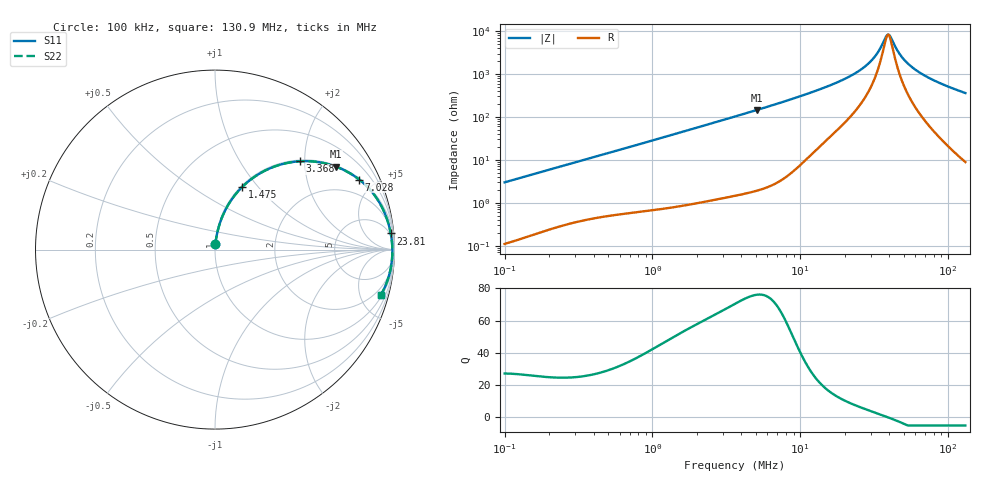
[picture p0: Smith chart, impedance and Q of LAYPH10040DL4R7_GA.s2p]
! LAYPH10040DL4R7_GA  S-PARAMETER MODEL  ( General Type )
! Model Generated by TAIYO YUDEN Corporation (http://www.ty-top.com)
! Version 1.0
! TAIYO YUDEN Control No. 180920NI43SB-FBB
! Copyright(c) 2018 TAIYO YUDEN CO.,LTD. All Rights Reserved.
! Product Description (link to TY-COMPAS)
! https://ds.yuden.co.jp/TYCOMPAS/or/detail?pn=LAYPH10040DL4R7NGA&u=M
! Products Name : Inductors
! Characteristics :
!  Inductance : 4.7 uH , SRF(min) : -Hz , DC Resistance(max) : 0.025 Ohm
!  Rated Current : Saturation :5.2 A , Temp Rise : 2.7 A (25 degC)
!  Case Size : 10.1 x 10.0 / 0.398 x 0.394 [mm/inch] , Thickness : 4 / 0.157 [mm/inch]
!  (Conditions: Temperature = 25 degC , DC Bias Current/Voltage = 0A / 0V)
! External Node Assignments :
!  1  o---GGG---o  2
! GND o---------o GND
! Frequency Range : 0.1MHz  -  130.914307MHz  [ 402 STEP ]
# MHz S RI R 50
! Freq[MHz].  S11 Real  S11 Imag  S21 Real  S21 Imag  S12 Real  S12 Imag  S22 Real  S22 Imag
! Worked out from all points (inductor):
!   401 points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, 100 kHz to 130.9 MHz, reference 50 ohm
!   read as one part in series: L = 4.73 uH near 103.7 kHz
!   highest Q = 76.1 at 5.088 MHz (marker M1), where L = 4.53 uH
!   self-resonance near 38.65 MHz
!   S11 on the Smith chart (normalised r, x): 100 kHz: 1.00, +0.06; 1.475 MHz: 1.02, +0.83; 3.368 MHz: 1.03, +1.90; 7.028 MHz: 1.06, +4.08; 23.81 MHz: 4, +21; 130.9 MHz: 1.18, -7.19
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0.1  0.00198 0.0298  0.998 -0.0298  0.998 -0.0298  0.00198 0.0298
0.332733  0.0128 0.0946  0.9872 -0.0946  0.9872 -0.0946  0.0128 0.0946
0.623493  0.0354 0.17  0.9646 -0.17  0.9646 -0.17  0.0354 0.17
1.10711  0.0941 0.2809  0.9059 -0.2809  0.9059 -0.2809  0.0941 0.2809
1.475265  0.152 0.3494  0.848 -0.3494  0.848 -0.3494  0.152 0.3494
2.189296  0.2782 0.4398  0.7218 -0.4398  0.7218 -0.4398  0.2782 0.4398
3.367625  0.4743 0.4921  0.5257 -0.4921  0.5257 -0.4921  0.4743 0.4921
3.683715  0.5191 0.4926  0.4809 -0.4926  0.4809 -0.4926  0.5191 0.4926
5.088039  0.6752 0.4618  0.3248 -0.4618  0.3248 -0.4618  0.6752 0.4618
7.027727  0.803 0.3905  0.197 -0.3905  0.197 -0.3905  0.803 0.3905
12.03896  0.9271 0.2423  0.0729 -0.2423  0.0729 -0.2423  0.9271 0.2423
17.86583  0.9653 0.1479  0.0347 -0.1479  0.0347 -0.1479  0.9653 0.1479
23.80689  0.9792 0.09  0.0208 -0.09  0.0208 -0.09  0.9792 0.09
27.48163  0.9835 0.0633  0.0165 -0.0633  0.0165 -0.0633  0.9835 0.0633
30.60534  0.9857 0.044  0.0143 -0.044  0.0143 -0.044  0.9857 0.044
34.08411  0.9872 0.025  0.0128 -0.025  0.0128 -0.025  0.9872 0.025
37.95831  0.988 0.00615  0.012 -0.00615  0.012 -0.00615  0.988 0.00615
40.05754  0.9882 -0.00326  0.0118 0.00326  0.0118 0.00326  0.9882 -0.00326
48.79793  0.9873 -0.0382  0.0127 0.0382  0.0127 0.0382  0.9873 -0.0382
59.44544  0.9839 -0.0746  0.0161 0.0746  0.0161 0.0746  0.9839 -0.0746
83.59406  0.9697 -0.1445  0.0303 0.1445  0.0303 0.1445  0.9697 -0.1445
130.9143  0.9228 -0.2548  0.0772 0.2548  0.0772 0.2548  0.9228 -0.2548
